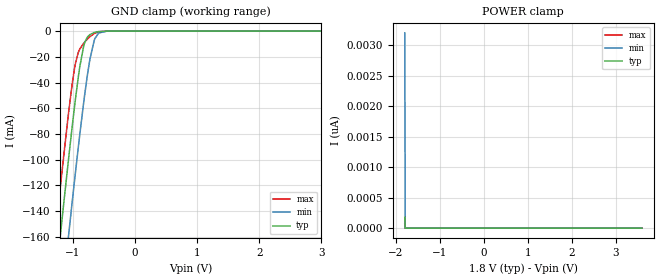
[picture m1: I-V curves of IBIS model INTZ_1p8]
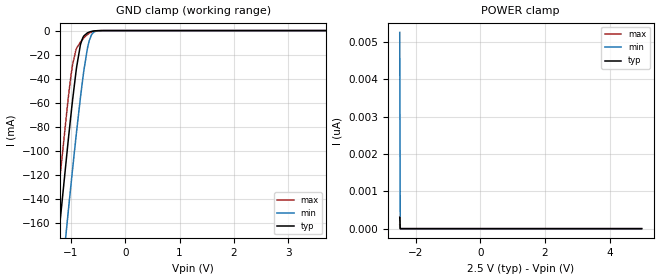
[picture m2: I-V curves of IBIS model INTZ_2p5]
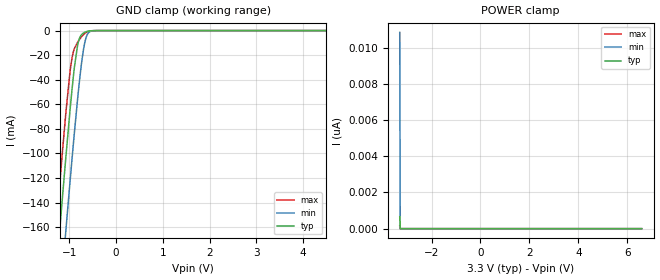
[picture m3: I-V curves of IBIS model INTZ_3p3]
|Texas Instruments Incorporated
| Low Voltage 4-channel I2C and SMbus Switch With Interrupt Logic and Reset
| Functions
| part#   Digital Voltage Range   Package-type   #pins
| TCA9545APWR   1.65V - 5.5V   TSSOP   20
[IBIS Ver]   4.1
[File name]   tca9545a.ibs
[File Rev]   1.0
[Date]   02/24/2014
[Source]
| Texas Instruments Incorporated.
| 12500 TI Blvd
| Dallas, TX -75243
[Notes]   Revision History:
| Rev 1.0: 02/24/2014
| - Initial version of the model
| - Model generated from simulations in TISPICE
| - C_comp although listed in numerical order of value are
|   obtained from varying PVT conditions. For PVT conditions for
|   each specific value refer the buffer description under
|   respective [Model]. IBIS model user is responsible for using
|   appropriate C_comp to simulate for Signal Integrity.
| - Warnings regarding combined/Non-monotonicity of various models have been
|   reviewd and considered minor and can be ignored.
| - Model names with a trailing _1p8 contains the model for 1.8V operation.
|   Model names with a trailing _2p5 contains the model for 2.5V operation.
|   Model names with a trailing _3p3 contains the model for 3.3V operation.
|   Model names with a trailing _5p0 contains the model for 5.0V operation.
[Disclaimer]
| This model is designed as an aid for customers of Texas Instruments.
| TI and its licensors and suppliers make no warranties, either expressed
| or implied, with respect to this  model, including the warranties of
| merchantability or fitness for a particular purpose. The model is
| provided solely on an "as is" basis. The entire risk as to its quality
| and performance is with the customer.
[Copyright]
 (C) Copyright 2014 Texas Instruments Incorporated.All rights reserved.
|   Device
[Component]   TCA9545A
[Manufacturer]   TI
[Package]
|   typ   min   max
R_pkg   0.129   0.115   0.141
L_pkg   3.095nH   2.582nH   3.694nH
C_pkg   0.529pF   0.443pF   0.631pF
[Pin]  signal_name   model_name   R_pin   L_pin   C_pin
1   A0   INTZ   0.1316   3.6895nH   0.63069pF
2   A1   INTZ   0.13599   3.37564nH   0.60133pF
3   RESTB   INTZ   0.13998   3.13062nH   0.50835pF
4   INT0   INTZ   0.1236   2.71161nH   0.46158pF
5   SD0   NC   0.11457   2.58287nH   0.4434pF
6   SC0   NC   0.11463   2.58513nH   0.44361pF
7   INT1   INTZ   0.12381   2.71917nH   0.46207pF
8   SD1   NC   0.14035   3.14662nH   0.51063pF
9   SC1   NC   0.13143   3.32932nH   0.59951pF
10   GND   GND   0.12987   3.67174nH   0.62362pF
11   INT2   INTZ   0.13131   3.69387nH   0.62714pF
12   SD2   NC   0.13189   3.33453nH   0.60249pF
13   SC2   NC   0.14054   3.14663nH   0.51179pF
14   INT3   INTZ   0.12397   2.72174nH   0.46221pF
15   SD3   NC   0.11469   2.58618nH   0.44359pF
16   SC3   NC   0.11452   2.58209nH   0.44334pF
17   INTB   INTZ_OP   0.12345   2.70908nH   0.46143pF
18   SCL   SCL   0.13978   3.13072nH   0.50728pF
19   SDA   SDA   0.13373   3.35743nH   0.60248pF
20   VCC   POWER   0.13135   3.68613nH   0.6287pF
|   Model Selectors
[Model Selector]  SDA
SDA_5p0   SDA buffer at 5.0V operation
SDA_3p3   SDA buffer at 3.3V operation
SDA_2p5   SDA buffer at 2.5V operation
SDA_1p8   SDA buffer at 1.8V operation
[Model Selector]  SCL
SCL_5p0   SCL buffer at 5.0V operation
SCL_3p3   SCL buffer at 3.3V operation
SCL_2p5   SCL buffer at 2.5V operation
SCL_1p8   SCL buffer at 1.8V operation
[Model Selector]  INTZ_OP
INTZ_OP_5p0   INTZ_OP buffer at 5.0V operation
INTZ_OP_3p3   INTZ_OP buffer at 3.3V operation
INTZ_OP_2p5   INTZ_OP buffer at 2.5V operation
INTZ_OP_1p8   INTZ_OP buffer at 1.8V operation
[Model Selector]  INTZ
INTZ_5p0   Input buffer at 5.0V operation
INTZ_3p3   Input buffer at 3.3V operation
INTZ_2p5   Input buffer at 2.5V operation
INTZ_1p8   Input buffer at 1.8V operation
| Models and submodels in the file (16): INTZ_1p8 (Input), INTZ_2p5 (Input), INTZ_3p3 (Input), INTZ_5p0 (Input), INTZ_OP_1p8 (Open_drain), INTZ_OP_2p5 (Open_drain), INTZ_OP_3p3 (Open_drain), INTZ_OP_5p0 (Open_drain), SCL_1p8 (Input), SCL_2p5 (Input), SCL_3p3 (Input), SCL_5p0 (Input), SDA_1p8 (I/O_open_drain), SDA_2p5 (I/O_open_drain), SDA_3p3 (I/O_open_drain), SDA_5p0 (I/O_open_drain)
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|   Model
[Model]   INTZ_1p8
Model_type   Input
Vinl = 0.54
Vinh = 1.26
|   typ   min   max
C_comp   1.378pF   1.292pF   1.466pF
[Voltage Range]   1.8   1.65   1.95
[Temperature Range]   27   125   -40
[Power Clamp Reference]   1.8   1.65   1.95
[GND Clamp Reference]   -0   -0   -0
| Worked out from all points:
|   GND clamp passes 1 mA (typ) near -0.65 V on its own axis
[GND Clamp]
|   Voltage   I(typ)   I(min)   I(max)
-1.8V     -444.5mA   -504.4mA   -407.1mA
-1.438V   -270.2mA   -330.8mA   -232.3mA
-1.222V   -168.5mA   -229.1mA   -130.8mA
-1.184V   -151.1mA   -211.6mA   -113.6mA
-1.071V   -100.1mA   -159.8mA   -64.28mA
-968.4mV  -56.83mA   -114.3mA   -27.68mA
-887.4mV  -27.43mA   -79.99mA   -13.89mA
-811.8mV  -9.407mA   -50.31mA   -8.666mA
-725.4mV  -2.729mA   -21.86mA   -4.347mA
-644.4mV  -935.9uA   -5.718mA   -1.642mA
-450mV    -25.03uA   -60uA      -30.72uA
3.595V    0A         0A         0A
[POWER Clamp]
|   Voltage   I(typ)   I(min)   I(max)
-1.8V     179.4pA    3.2nA      72.27pA
-1.789V   0A         0A         0A
-1.784V   0A         0A         0A
3.595V    0A         0A         0A
|   Model
[Model]   INTZ_2p5
Model_type   Input
Vinl = 0.75
Vinh = 1.75
|   typ   min   max
C_comp   1.378pF   1.292pF   1.466pF
[Voltage Range]   2.5   2.3   2.7
[Temperature Range]   27   125   -40
[Power Clamp Reference]   2.5   2.3   2.7
[GND Clamp Reference]   -0   -0   -0
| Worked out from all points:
|   GND clamp passes 1 mA (typ) near -0.65 V on its own axis
[GND Clamp]
|   Voltage   I(typ)   I(min)   I(max)
-2.5V     -787mA     -845.5mA   -750.7mA
-1.48V    -290.1mA   -350.6mA   -252.3mA
-1.285V   -197.8mA   -258.4mA   -159.9mA
-1.218V   -166.4mA   -226.9mA   -128.7mA
-1.052V   -92.02mA   -151.4mA   -56.8mA
-970mV    -57.47mA   -115mA     -28.12mA
-910mV    -34.93mA   -89.36mA   -16.29mA
-827.5mV  -12.06mA   -56.22mA   -9.593mA
-692.5mV  -1.8mA     -13.74mA   -3.073mA
-610mV    -552.2uA   -2.69mA    -947uA
-475mV    -43.19uA   -107.4uA   -55.89uA
4.992V    0A         0A         0A
[POWER Clamp]
|   Voltage   I(typ)   I(min)   I(max)
-2.5V     306.4pA    5.259nA    105.1pA
-2.485V   0A         0A         0A
-2.478V   0A         0A         0A
4.992V    0A         0A         0A
|   Model
[Model]   INTZ_3p3
Model_type   Input
Vinl = 0.99
Vinh = 2.31
|   typ   min   max
C_comp   1.378pF   1.292pF   1.466pF
[Voltage Range]   3.3   3   3.6
[Temperature Range]   27   125   -40
[Power Clamp Reference]   3.3   3   3.6
[GND Clamp Reference]   -0   -0   -0
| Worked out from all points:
|   GND clamp passes 1 mA (typ) near -0.65 V on its own axis
[GND Clamp]
|   Voltage   I(typ)   I(min)   I(max)
-3.3V     -1.182A    -1.239A    -1.146A
-1.34V    -223.5mA   -284.2mA   -185.6mA
-1.28V    -195.6mA   -256.3mA   -157.7mA
-1.211V   -163.4mA   -223.9mA   -125.7mA
-1.082V   -105.1mA   -164.9mA   -69mA
-943.8mV  -47.25mA   -103.7mA   -21.79mA
-825mV    -11.6mA    -55.27mA   -9.442mA
-735.9mV  -3.119mA   -24.84mA   -4.801mA
-656.7mV  -1.116mA   -7.317mA   -1.956mA
-577.5mV  -319uA     -1.25mA    -520.2uA
-409.2mV  -9.659uA   -23.55uA   -10.74uA
6.59V     0A         0A         0A
[POWER Clamp]
|   Voltage   I(typ)   I(min)   I(max)
-3.3V     664pA      10.84nA    162.7pA
-3.28V    0A         0A         0A
-3.27V    0A         0A         0A
6.59V     0A         0A         0A
